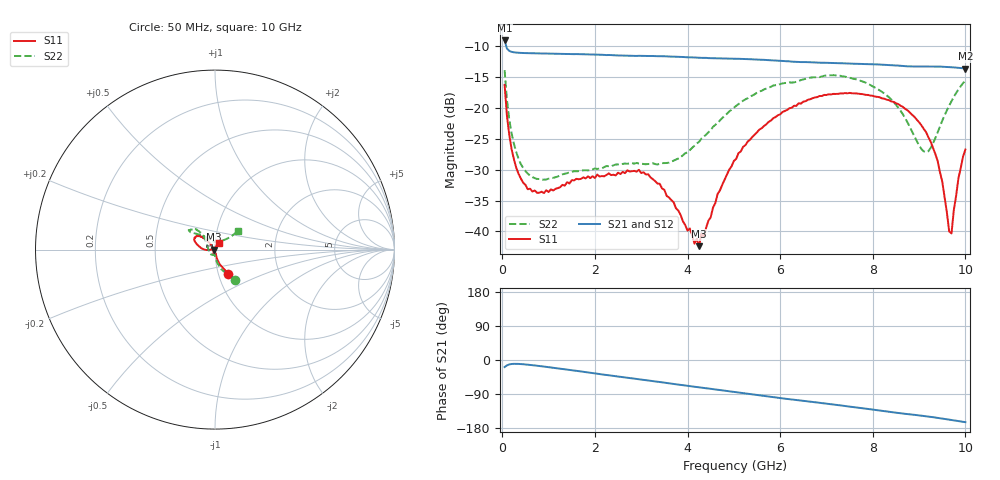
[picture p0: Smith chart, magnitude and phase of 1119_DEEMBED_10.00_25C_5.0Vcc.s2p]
!Hittite Microwave Corp.
!Digital Attenuator/PhaseShifter Rev 1.4.0
!Filename: C:\DATA\DATA\1119_DEEMBED_10.00_25C_5.0Vcc.s2p
!VNA ID: Agilent Technologies,N5224A,MY51441122,A.10.45.03
!Device type:
!2 Port Calibration.
!Temp(C): 25
!Lot Number:
!Serial Number:
!Operator:
!Misc:
!Attenuator:  10.000
# GHZ S DB R 50.0
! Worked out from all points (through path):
!   200 points, 50 MHz to 10 GHz, reference 50 ohm
!   highest |S21| = -9.15 dB at 50 MHz (marker M1); lowest = -13.7 dB at 10 GHz (marker M2)
!   group delay of S21, straight-line fit = 44 ps
!   lowest |S11| = -42.4 dB at 4.25 GHz (marker M3), VSWR 1.02, Z = 49.2 - j0.0652 ohm
!   |S11| at or under -10 dB: start of sweep to end of sweep
!   |S22| runs from -31.6 to -13.9 dB; largest |S21 - S12| = 0.0009
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0.05  -16.33 -61.2  -9.15 -18.6  -9.15 -18.6  -13.95 -57.1
0.1  -21.29 -72.2  -10.45 -14.2  -10.45 -14.2  -18.71 -72.2
0.2  -26.67 -78.0  -10.99 -10.6  -10.99 -10.6  -24.12 -82.7
0.35  -30.67 -78.6  -11.14 -10.3  -11.14 -10.3  -28.24 -88.1
0.55  -33.18 -80.8  -11.20 -12.3  -11.20 -12.3  -30.66 -92.6
1.75  -31.26 -102.2  -11.38 -31.1  -11.38 -31.2  -30.12 -110.2
2.95  -30.04 -102.9  -11.63 -50.6  -11.64 -50.6  -29.02 -147.8
3.4  -32.29 -109.3  -11.69 -58.1  -11.70 -58.1  -29.06 -168.6
4.25  -42.37 -175.0  -11.94 -72.2  -11.96 -72.3  -25.51 147.1
4.65  -33.94 133.2  -12.03 -78.5  -12.05 -78.5  -22.45 134.6
5.05  -28.28 128.9  -12.11 -84.8  -12.13 -84.9  -19.71 129.9
5.75  -22.31 133.1  -12.33 -96.4  -12.35 -96.5  -16.77 132.4
6.7  -18.48 141.0  -12.68 -110.7  -12.69 -110.7  -15.11 140.1
7.65  -17.70 153.0  -12.92 -125.3  -12.93 -125.3  -15.43 144.7
8.35  -18.79 160.3  -13.12 -136.6  -13.12 -136.6  -18.33 135.8
9.15  -23.94 178.8  -13.36 -148.4  -13.37 -148.4  -27.20 85.8
9.400001  -28.60 -176.2  -13.37 -152.6  -13.38 -152.7  -24.03 52.2
9.5  -31.92 179.9  -13.39 -154.5  -13.40 -154.6  -22.11 45.0
9.65  -39.99 139.7  -13.45 -157.4  -13.47 -157.3  -19.67 40.1
9.7  -40.31 108.1  -13.48 -158.3  -13.49 -158.3  -18.95 39.3
9.85  -31.40 63.9  -13.57 -161.2  -13.57 -161.2  -17.07 39.2
10  -26.77 59.3  -13.68 -164.1  -13.68 -164.1  -15.59 39.6
